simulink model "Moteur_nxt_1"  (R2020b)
settings: Solver=FixedStepAuto  StartTime=0.0  StopTime=inf  RelTol=1e-3  EnableMultiTasking=on
libraries: arduinolib x3, simulink x1

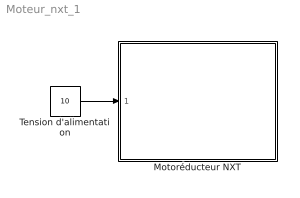
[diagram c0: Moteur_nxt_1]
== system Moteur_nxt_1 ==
  Motoréducteur NXT : Subsystem
  Tension d'alimentation : Constant  Value=10
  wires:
  Tension d'alimentation/1 -> Motoréducteur NXT/1(U)

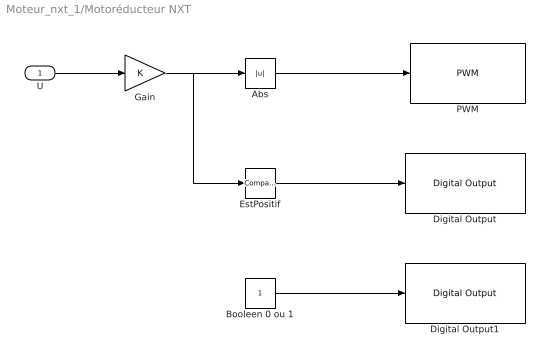
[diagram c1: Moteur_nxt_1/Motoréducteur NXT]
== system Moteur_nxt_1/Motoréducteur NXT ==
  U : Inport
  Abs : Abs
  Booleen 0 ou 1 : Constant
  Digital Output : arduinolib/Digital Output  pinNumber=3  Direction=output  blockPlatform=arduino
  Digital Output1 : arduinolib/Digital Output  pinNumber=3  Direction=output  blockPlatform=arduino
  EstPositif : simulink/Logic and Bit Operations/Compare To Zero  relop=>  OutDataTypeStr=boolean
  Gain : Gain
  PWM : arduinolib/PWM  pinNumber=3  frequencyType=Default  desiredFrequency=490.2  achievableFrequency=490.2
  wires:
  EstPositif/1 -> Digital Output/1
  U/1 -> Gain/1
  Gain/1 -> EstPositif/1, Abs/1
  Abs/1 -> PWM/1
  Booleen 0 ou 1/1 -> Digital Output1/1
